VAR_GLOBAL
	
//datapoints SLAVE -> MASTER (monitoring direction)
	(* Input *)

	(* Output *)
	
	(* Memory *)
	
	(* Data *)
		(*Single points*)
			// bSlaveToMaster
			bSlaveToMaster 			: BOOL;		// obj addr: 10 - M_SP_NA_1
			nSIQ_bSlaveToMaster 	: BYTE;		// value and quality descriptor
			eSPI_bSlaveToMaster		: E_IEC870_5_101SPI;// value as enum type
			nQDS_bSlaveToMaster		: BYTE;		// quality descriptor only
		
		(*Bitstrings*)
			// nBitstring
			nBitstring 				: DWORD;	// obj addr: 11 - M_BO_TB_1
			nQDS_nBitstring			: BYTE;		// quality descriptor
		
		(*Measurement value*)
			// nMeasurementValue - scaled value
			nMeasurementValue 		: INT;		// obj addr: 12 - M_ME_NB_1
			nQDS_nMeasurementValue 	: BYTE;		// quality descriptor
			
			// fMeasurementValue - short floating point value
			fMeasurementValue 		: REAL;		// obj addr: 13 - M_ME_NC_1
			nQDS_fMeasurementValue 	: BYTE;		// quality descriptor
			
		(*Integrated totals*)
			// nCounter
			nBCR_nCounter			: DWORD:=0;	// obj addr: 200 - M_IT_NA_1
			nBCR_QDS				: BYTE;		// quality descriptor
			
			
//datapoints MASTER -> SLAVE (control direction)
	(* Input *)

	(* Output *)
	
	(* Memory *)
	
	(* Data *)
		(*Single Commands*)
			// bMasterToSlave
			bMasterToSlave 			: BOOL;		// obj addr: 101 - C_SC_NA_1
			nSCO_bMasterToSlave 	: BYTE;		// command value and qualifier 
			eSCS_bMasterToSlave		: E_IEC870_5_101SCS;// command value as enum type
			eQU_bMasterToSlave		: E_IEC870_5_101QU;// command qualifier only

//other variables
	(* Slock sync*)
		tActTime					: T_CP56Time2a;	// actual time
		bDSTime						: BOOL;			// daylight saving time
END_VAR
